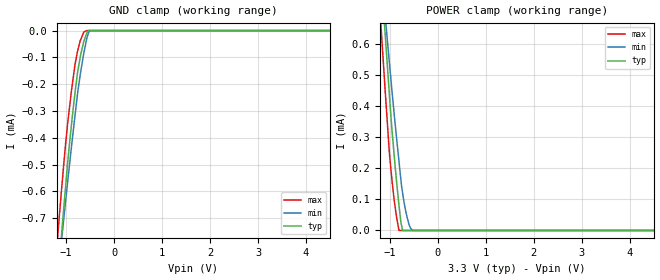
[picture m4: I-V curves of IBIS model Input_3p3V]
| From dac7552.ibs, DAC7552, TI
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|   Model   - Input_3p3V
[Model]   Input_3p3V
Model_type   Input
Vinl = 0.99
Vinh = 2.31
|   typ   min   max
|   (nom PVT)   (Fast PVT)   (slow PVT)
|Average
C_comp   1.795e-13   1.762e-13   1.858e-13
| Where   nom  PVT is  Nominal Process, 3.3V, 25C
|   Fast PVT is Strong Process, 3.6V, -40C
|   Slow PVT is Weak Process, 3.0V, 105C
[model spec]
Vinl   0.99   0.9   1.08
Vinh   2.31   2.1   2.52
[Voltage Range]   3.3   3   3.6
|Ambient Temperature   25   105   -40
|Junction Temperature
[Temperature Range]   25   105   -40
[Power Clamp Reference]   3.3   3   3.6
[GND Clamp Reference]   0   0   0
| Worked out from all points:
|   GND clamp passes 1 mA (typ) near -1.20 V on its own axis
|   POWER clamp passes 1 mA (typ) near -1.26 V on its own axis
[GND Clamp]
|   Voltage   I(typ)   I(min)   I(max)
-3.3V     -6.099mA   -4.811mA   -6.201mA
-1.168V   -921.1uA   -908.9uA   -750.3uA
-1.09V    -749.5uA   -772.3uA   -581.4uA
-1.069V   -705uA     -737.3uA   -539.7uA
-963.6mV  -484.7uA   -556.8uA   -339.7uA
-816mV    -234.4uA   -319.1uA   -128.7uA
-765.6mV  -161.7uA   -241.4uA   -80.2uA
-696.3mV  -89.29uA   -154uA     -33.63uA
-636mV    -43.51uA   -89.32uA   -7.488uA
-573mV    -12.06uA   -32.46uA   0A
-510mV    0A         0A         0A
6.6V      0A         0A         0A
[POWER Clamp]
|   Voltage   I(typ)   I(min)   I(max)
-3.3V     5.989mA    4.71mA     6.109mA
-1.205V   875.5uA    874.3uA    703.5uA
-1.155V   760.1uA    787uA      585.3uA
-1.1V     636.9uA    693.8uA    455.7uA
-1.082V   596.4uA    663.1uA    413.8uA
-1.01V    437.3uA    540.5uA    250uA
-956.4mV  323.8uA    448.5uA    161.2uA
-808.8mV  78.96uA    220.3uA    0A
-732.6mV  0A         118.7uA    0A
-642mV    0A         42.68uA    0A
-525mV    0A         0A         0A
6.6V      0A         0A         0A
